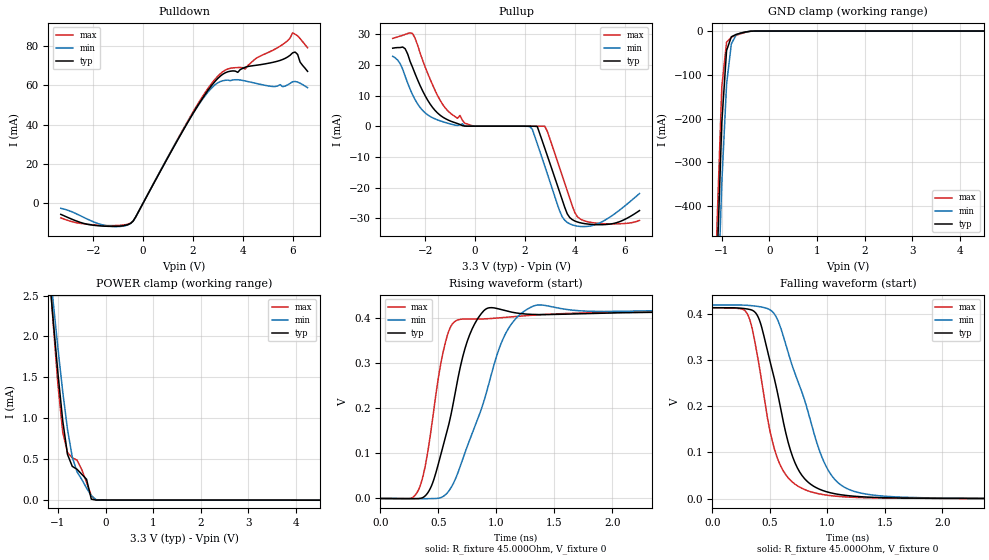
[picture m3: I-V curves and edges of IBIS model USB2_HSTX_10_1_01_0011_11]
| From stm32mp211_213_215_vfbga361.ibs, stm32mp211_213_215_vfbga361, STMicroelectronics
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[Model] USB2_HSTX_10_1_01_0011_11
Model_type   Output
Polarity   Non-Inverting
Enable   Active-High
C_comp   8.036pF   7.631pF   8.569pF
Vmeas = 200.000mV
Vref = 200.000mV
Rref = 45Ohms
Cref = 0pF
[Model Spec]
Vmeas   200.000mV   200.000mV   200.000mV
Vref   200.000mV   200.000mV   200.000mV
| This model is not intended for timing simulations.
| Warnings about Cref, Vref & Rref can be ignored
[Temperature Range]   25.000   125.000   -40.000
[Voltage Range]   3.300V   3.070V   3.630V
[GND Clamp Reference]   0.00V   0.00V   0.00V
[Pulldown Reference]   0.00V   0.00V   0.00V
[POWER Clamp Reference]   3.300V   3.070V   3.630V
[Pullup Reference]   3.300V   3.070V   3.630V
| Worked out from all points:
|   slope of the pulldown table from 0 to 0.495 V, typ, clamps not added: 42.6 ohm
|   GND clamp passes 1 mA (typ) near -0.43 V on its own axis
|   POWER clamp passes 1 mA (typ) near -0.91 V on its own axis
|   rising waveform, R_fixture 45.000Ohm, V_fixture 0: 20-80 % time 222ps typ, 324ps min, 152ps max; typ from 0 V to 0.413 V
|   falling waveform, R_fixture 45.000Ohm, V_fixture 0: 20-80 % time 242ps typ, 327ps min, 197ps max; typ from 0.413 V to 0 V
[GND Clamp]
-3.3V     -11.02A    -10.62A    -11.32A
-1.2V     -931.6mA   -1.049A    -855.7mA
-1.1V     -533.1mA   -671.7mA   -440.2mA
-1V       -209.4mA   -347mA     -127.3mA
-900mV    -44.44mA   -121.7mA   -25.6mA
-800mV    -13.15mA   -29.48mA   -14.15mA
-700mV    -7.742mA   -9.125mA   -9.769mA
-500mV    -2.127mA   -1.981mA   -2.894mA
-300mV    -19.47uA   -62.22uA   -13.76uA
6.6V      10.37uA    26.59uA    21.05uA
[Power Clamp]
-3.3V     3.206A     2.175A     4.855A
-1.2V     2.88mA     3.008mA    2.969mA
-1.1V     2.195mA    2.419mA    2.156mA
-1V       1.545mA    1.852mA    1.406mA
-900mV    969.9uA    1.324mA    831.4uA
-800mV    558.5uA    864.6uA    580.3uA
-700mV    412uA      525.9uA    517uA
-600mV    376.6uA    345uA      488.5uA
-400mV    254.2uA    146.6uA    216.8uA
-300mV    11.21uA    52.87uA    53.51uA
-100mV    94.86nA    985nA      361.1nA
6.6V      -2.721uA   -5.18uA    -3.077uA
[Pulldown]
-3.3V     -5.671mA   -2.581mA   -7.449mA
-1.6V     -11.64mA   -11.09mA   -11.31mA
-500mV    -10.25mA   -10.32mA   -10.1mA
1.9V      43.42mA    43.46mA    44.13mA
2.9V      62.15mA    60.37mA    63.26mA
3.4V      66.87mA    62.63mA    68.29mA
4.1V      69.19mA    62.19mA    68.26mA
4.5V      70.11mA    61.06mA    73.4mA
5.6V      73.12mA    59.29mA    80.76mA
6V        76.51mA    61.79mA    86.69mA
6.1V      76.9mA     61.92mA    85.99mA
6.6V      67.09mA    58.79mA    79.1mA
[Pullup]
-3.3V     25.51mA    22.87mA    28.71mA
-2.8V     25.33mA    16.38mA    30mA
-2.5V     19.21mA    10.28mA    30.27mA
-1.2V     2.603mA    1.31mA     6.11mA
-100mV    93.8uA     82.61uA    220.4uA
2.2V      68.65uA    -28.24uA   104.8uA
2.5V      -41.39uA   -5.658mA   83.49uA
2.9V      -9.472mA   -15.37mA   -1.562mA
3.5V      -23.92mA   -29.44mA   -16.02mA
3.8V      -29.68mA   -31.75mA   -23.35mA
4.4V      -31.68mA   -32.65mA   -30.79mA
6.6V      -27.44mA   -21.87mA   -30.63mA
[Ramp]
R_load=45.000Ohm
dV/dt_r   624.172mV/1.090ns  592.504mV/1.140ns  677.764mV/990.000ps
dV/dt_f   626.381mV/265.000ps  595.438mV/350.000ps  679.594mV/225.000ps
[Rising waveform]
R_fixture=45.000Ohm
V_fixture=0
0s        452.3nV    3.134uV    468nV
300ps     -354.4uV   -317.7uV   7.263mV
420ps     17.18mV    -365.6uV   121.4mV
520ps     95.95mV    1.919mV    297.1mV
600ps     174.9mV    20.16mV    376.8mV
750ps     348.3mV    116mV      397mV
940ps     421.7mV    258.7mV    397.7mV
1.11ns    413.1mV    378.3mV    401.2mV
1.36ns    406.6mV    427.8mV    406mV
9.9ns     413.1mV    419.1mV    412.8mV
[Falling waveform]
R_fixture=45.000Ohm
V_fixture=0
0s        412.6mV    418.6mV    412.3mV
310ps     409.6mV    417.6mV    396.7mV
410ps     385.7mV    414.9mV    283.8mV
540ps     258.8mV    398.9mV    107.5mV
650ps     130.9mV    323.5mV    48.16mV
720ps     77.02mV    269.7mV    31.28mV
960ps     17.69mV    85.69mV    9.02mV
1.17ns    6.826mV    21.97mV    3.649mV
1.66ns    1.343mV    3.211mV    915.5uV
9.9ns     13.78uV    31.08uV    3.882uV
